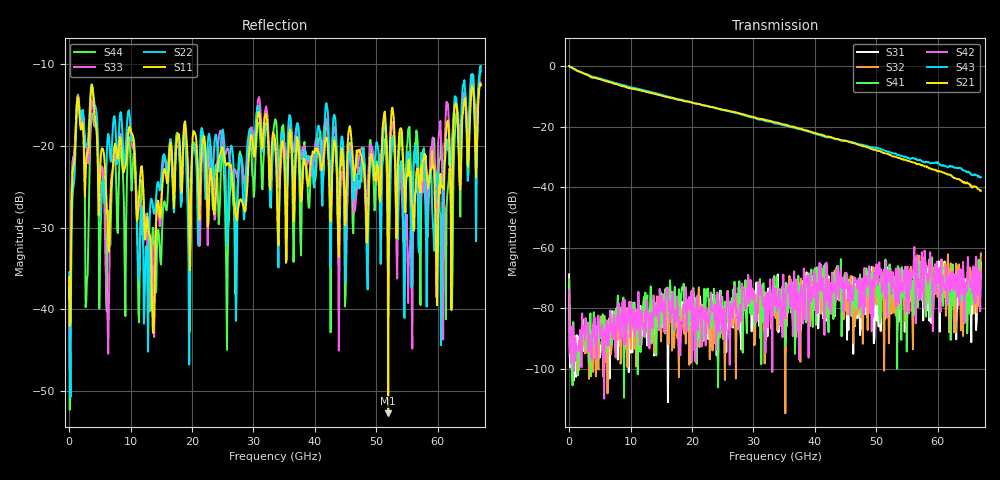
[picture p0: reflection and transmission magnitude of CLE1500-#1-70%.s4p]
!Keysight Technologies,N5247B,US50470101,A.16.20.02
!Date: Thursday, March 13, 2025 10:27:31
!Correction: S11(C  4-Port  )
!S12(C  4-Port  )
!S13(C  4-Port  )
!S14(C  4-Port  )
!S21(C  4-Port  )
!S22(C  4-Port  )
!S23(C  4-Port  )
!S24(C  4-Port  )
!S31(C  4-Port  )
!S32(C  4-Port  )
!S33(C  4-Port  )
!S34(C  4-Port  )
!S41(C  4-Port  )
!S42(C  4-Port  )
!S43(C  4-Port  )
!S44(C  4-Port  )
!S4P File: Measurements: <S11,S12,S13,S14>,
!<S21,S22,S23,S24>,
!<S31,S32,S33,S34>,
!<S41,S42,S43,S44>:
# Hz S  dB  R 50
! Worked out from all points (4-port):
!   601 points, 10 MHz to 67 GHz, reference 50 ohm
!   strongest paths, dB at 10 MHz, 16.76 GHz, 33.51 GHz, 50.25 GHz, 67 GHz:
!     S21: 0.0, -10.6, -18.5, -28.0, -41.1
!     S43: 0.0, -10.4, -18.9, -27.3, -36.7
!     S42: -74.1, -76.8, -79.0, -72.4, -68.2
!     S41: -70.6, -76.2, -80.2, -71.0, -69.3
!     S32: -70.5, -94.0, -81.8, -71.5, -61.9
!     S31: -68.8, -87.9, -77.5, -79.5, -64.9
!   lowest |S11| = -52.7 dB at 51.93 GHz (marker M1), VSWR 1.00, Z = 49.9 - j0.225 ohm
!   |S11| at or under -10 dB: start of sweep to end of sweep
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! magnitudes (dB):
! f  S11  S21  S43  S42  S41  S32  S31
! 10 MHz  -36.1  0.0  0.0  -74.1  -70.6  -70.5  -68.8
! 3.806 GHz  -12.8  -3.8  -3.5  -87.6  -92.0  -100.3  -95.2
! 6.262 GHz  -29.6  -5.1  -4.8  -92.1  -85.3  -108.1  -84.6
! 9.835 GHz  -17.6  -7.3  -6.9  -77.8  -82.6  -84.2  -89.3
! 12.51 GHz  -30.0  -8.5  -8.2  -87.3  -84.6  -88.1  -83.7
! 51.93 GHz  -52.7  -29.0  -28.3  -67.5  -81.0  -70.4  -79.7
! 67 GHz  -12.6  -41.1  -36.7  -68.2  -69.3  -61.9  -64.9
